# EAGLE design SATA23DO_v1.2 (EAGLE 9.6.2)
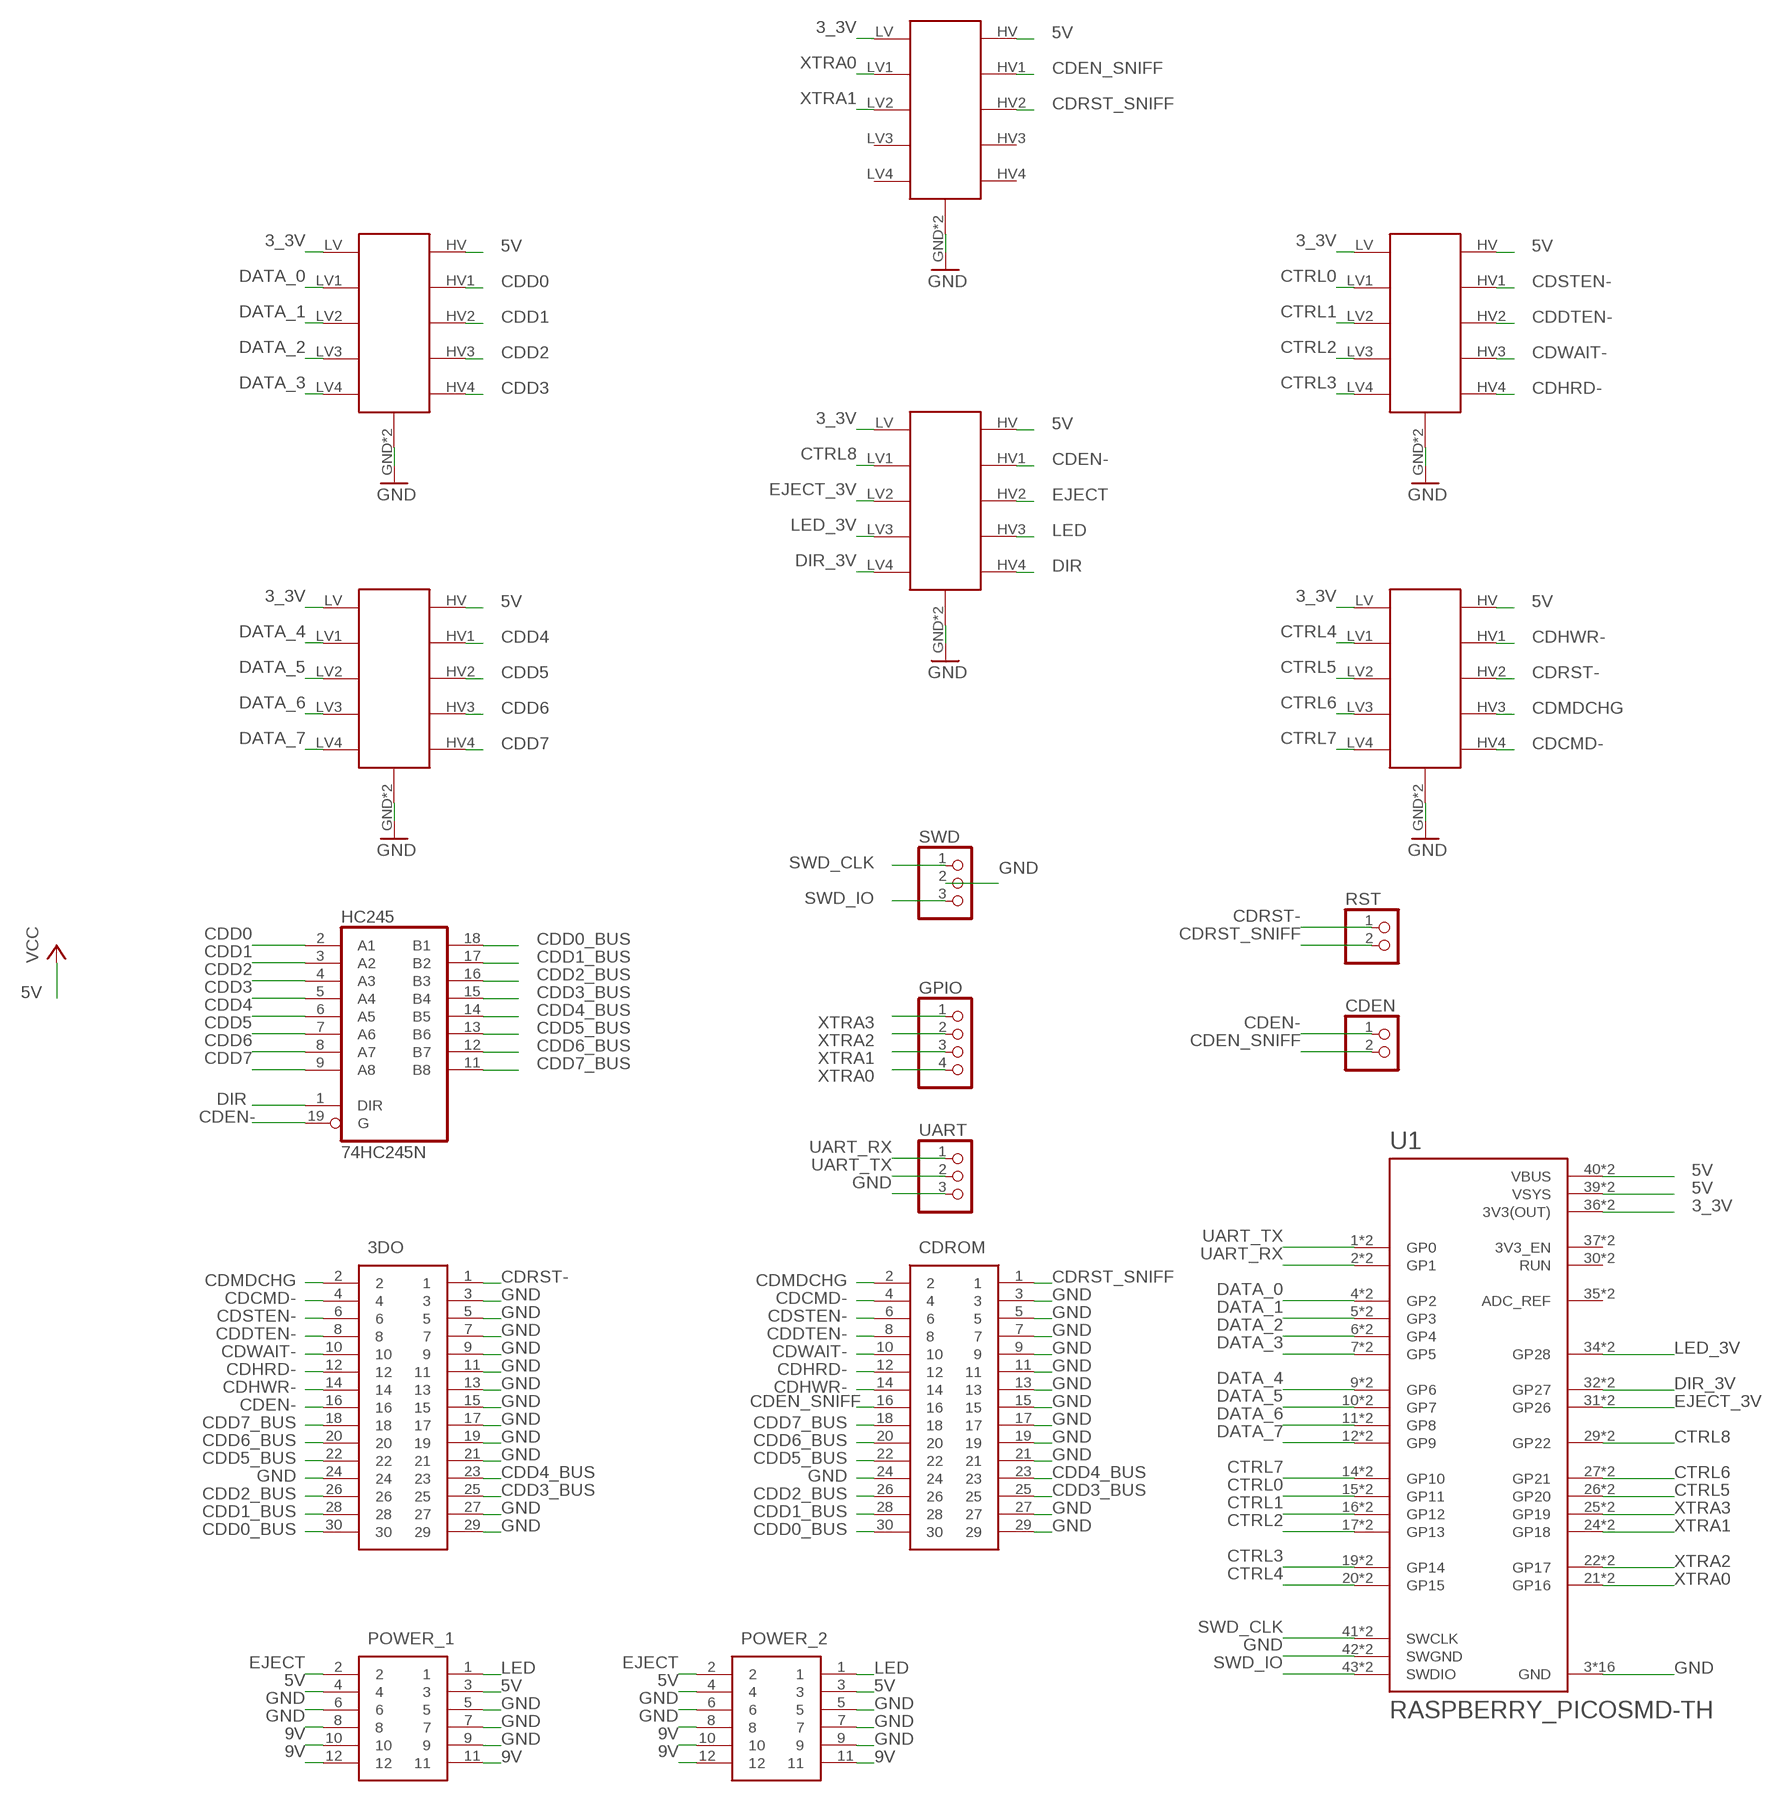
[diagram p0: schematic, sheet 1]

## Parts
3DO  52045-304530PIN_REVERSE  [30PINFFC125_REVERSE]
CDEN  PINHD-1X2  [1X02]
CDROM  52045-304530PIN_REVERSE  [30PINFFC125_REVERSE]
GPIO  PINHD-1X4  [1X04]
HC245  74HC245N  [DIL20]
POWER_1  39-53-2125  [39532125]
POWER_2  39-53-2125  [39532125]
RST  PINHD-1X2  [1X02]
SWD  PINHD-1X3  [1X03]
U1  RASPBERRY_PICOSMD-TH  [PICO-PKG]
U$1  4WAYS_LEVEL_SHIFTER  [4WAYS_LEVEL_SHIFTER]
U$5  4WAYS_LEVEL_SHIFTER  [4WAYS_LEVEL_SHIFTER]
U$6  4WAYS_LEVEL_SHIFTER  [4WAYS_LEVEL_SHIFTER]
U$7  4WAYS_LEVEL_SHIFTER  [4WAYS_LEVEL_SHIFTER]
U$8  4WAYS_LEVEL_SHIFTER  [4WAYS_LEVEL_SHIFTER]
U$9  4WAYS_LEVEL_SHIFTER  [4WAYS_LEVEL_SHIFTER]
UART  PINHD-1X3  [1X03]

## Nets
3_3V: U1.36(3V3(OUT)) U1.P$36(3V3(OUT)) U$1.LV U$5.LV U$6.LV U$7.LV U$8.LV U$9.LV
5V: POWER_1.3 POWER_1.4 POWER_2.3 POWER_2.4 U1.39(VSYS) U1.40(VBUS) U1.P$39(VSYS) U1.P$40(VBUS) U$1.HV U$5.HV U$6.HV U$7.HV U$8.HV U$9.HV ; supply symbol labelled VCC
9V: POWER_1.10 POWER_1.11 POWER_1.12 POWER_2.10 POWER_2.11 POWER_2.12
CDCMD-: 3DO.4 CDROM.4 U$7.HV4
CDD0: HC245.2(A1) U$6.HV1
CDD0_BUS: 3DO.30 CDROM.30 HC245.18(B1)
CDD1: HC245.3(A2) U$6.HV2
CDD1_BUS: 3DO.28 CDROM.28 HC245.17(B2)
CDD2: HC245.4(A3) U$6.HV3
CDD2_BUS: 3DO.26 CDROM.26 HC245.16(B3)
CDD3: HC245.5(A4) U$6.HV4
CDD3_BUS: 3DO.25 CDROM.25 HC245.15(B4)
CDD4: HC245.6(A5) U$5.HV1
CDD4_BUS: 3DO.23 CDROM.23 HC245.14(B5)
CDD5: HC245.7(A6) U$5.HV2
CDD5_BUS: 3DO.22 CDROM.22 HC245.13(B6)
CDD6: HC245.8(A7) U$5.HV3
CDD6_BUS: 3DO.20 CDROM.20 HC245.12(B7)
CDD7: HC245.9(A8) U$5.HV4
CDD7_BUS: 3DO.18 CDROM.18 HC245.11(B8)
CDDTEN-: 3DO.8 CDROM.8 U$8.HV2
CDEN-: 3DO.16 CDEN.1 HC245.19(G) U$9.HV1
CDEN_SNIFF: CDEN.2 CDROM.16 U$1.HV1
CDHRD-: 3DO.12 CDROM.12 U$8.HV4
CDHWR-: 3DO.14 CDROM.14 U$7.HV1
CDMDCHG: 3DO.2 CDROM.2 U$7.HV3
CDRST-: 3DO.1 RST.1 U$7.HV2
CDRST_SNIFF: CDROM.1 RST.2 U$1.HV2
CDSTEN-: 3DO.6 CDROM.6 U$8.HV1
CDWAIT-: 3DO.10 CDROM.10 U$8.HV3
CTRL0: U1.15(GP11) U1.P$15(GP11) U$8.LV1
CTRL1: U1.16(GP12) U1.P$16(GP12) U$8.LV2
CTRL2: U1.17(GP13) U1.P$17(GP13) U$8.LV3
CTRL3: U1.19(GP14) U1.P$19(GP14) U$8.LV4
CTRL4: U1.20(GP15) U1.P$20(GP15) U$7.LV1
CTRL5: U1.26(GP20) U1.P$26(GP20) U$7.LV2
CTRL6: U1.27(GP21) U1.P$27(GP21) U$7.LV3
CTRL7: U1.14(GP10) U1.P$14(GP10) U$7.LV4
CTRL8: U1.29(GP22) U1.P$29(GP22) U$9.LV1
DATA_0: U1.4(GP2) U1.P$4(GP2) U$6.LV1
DATA_1: U1.5(GP3) U1.P$5(GP3) U$6.LV2
DATA_2: U1.6(GP4) U1.P$6(GP4) U$6.LV3
DATA_3: U1.7(GP5) U1.P$7(GP5) U$6.LV4
DATA_4: U1.9(GP6) U1.P$9(GP6) U$5.LV1
DATA_5: U1.10(GP7) U1.P$10(GP7) U$5.LV2
DATA_6: U1.11(GP8) U1.P$11(GP8) U$5.LV3
DATA_7: U1.12(GP9) U1.P$12(GP9) U$5.LV4
DIR: HC245.1(DIR) U$9.HV4
DIR_3V: U1.32(GP27) U1.P$32(GP27) U$9.LV4
EJECT: POWER_1.2 POWER_2.2 U$9.HV2
EJECT_3V: U1.31(GP26) U1.P$31(GP26) U$9.LV2
GND: 3DO.3 3DO.5 3DO.7 3DO.9 3DO.11 3DO.13 3DO.15 3DO.17 3DO.19 3DO.21 3DO.24 3DO.27 3DO.29 CDROM.3 CDROM.5 CDROM.7 CDROM.9 CDROM.11 CDROM.13 CDROM.15 CDROM.17 CDROM.19 CDROM.21 CDROM.24 CDROM.27 CDROM.29 POWER_1.5 POWER_1.6 POWER_1.7 POWER_1.8 POWER_1.9 POWER_2.5 POWER_2.6 POWER_2.7 POWER_2.8 POWER_2.9 SWD.2 U1.3(GND) U1.8(GND) U1.13(GND) U1.18(GND) U1.23(GND) U1.28(GND) U1.33(GND) U1.38(GND) U1.42(SWGND) U1.P$3(GND) U1.P$8(GND) U1.P$13(GND) U1.P$18(GND) U1.P$23(GND) U1.P$28(GND) U1.P$33(GND) U1.P$38(GND) U1.P$42(SWGND) U$1.GND U$1.GND_1(GND) U$5.GND U$5.GND_1(GND) U$6.GND U$6.GND_1(GND) U$7.GND U$7.GND_1(GND) U$8.GND U$8.GND_1(GND) U$9.GND U$9.GND_1(GND) UART.3
LED: POWER_1.1 POWER_2.1 U$9.HV3
LED_3V: U1.34(GP28) U1.P$34(GP28) U$9.LV3
SWD_CLK: SWD.1 U1.41(SWCLK) U1.P$41(SWCLK)
SWD_IO: SWD.3 U1.43(SWDIO) U1.P$43(SWDIO)
UART_RX: U1.2(GP1) U1.P$2(GP1) UART.1
UART_TX: U1.1(GP0) U1.P$1(GP0) UART.2
XTRA0: GPIO.4 U1.21(GP16) U1.P$21(GP16) U$1.LV1
XTRA1: GPIO.3 U1.24(GP18) U1.P$24(GP18) U$1.LV2
XTRA2: GPIO.2 U1.22(GP17) U1.P$22(GP17)
XTRA3: GPIO.1 U1.25(GP19) U1.P$25(GP19)
Unconnected: U1.30(RUN) U1.35(ADC_REF) U1.37(3V3_EN) U1.P$30(RUN) U1.P$35(ADC_REF) U1.P$37(3V3_EN) U$1.HV3 U$1.HV4 U$1.LV3 U$1.LV4

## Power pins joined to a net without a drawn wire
5V: HC245.20(VCC)
GND: HC245.10(GND)

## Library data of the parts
3DO CDROM = SamacSys_Parts:52045-3045
CDEN RST = Connector:PINHD-1X2: PIN HEADER; CATEGORY: CONNECTOR; SUB-CATEGORY: PIN-HEADER
GPIO = Connector:PINHD-1X4: PIN HEADER; CATEGORY: CONNECTOR; SUB-CATEGORY: PIN-HEADER
HC245 = 74xx-eu:74*245: Octal BUS TRANSCEIVER, 3-state
POWER_1 POWER_2 = SamacSys_Parts:39-53-2125: Molex FFC/FPC THROUGH HOLE Series 1.25mm Pitch 12 Way 1 Row Straight Through Hole Female FPC Connector Source: Datasheet; ALLIED_NUMBER: 70373145; DESCRIPTION: Molex FFC/FPC THROUGH HOLE Series 1.25mm Pitch 12 Way 1 Row Straight Through Hole Female FPC Connector; HEIGHT: 10mm; MANUFACTURER_NAME: Molex; MANUFACTURER_PART_NUMBER: 39-53-2125; RS_PART_NUMBER: 5427084; RS_PRICE-STOCK: https://uk.rs-online.com/web/p/products/5427084
SWD UART = Connector:PINHD-1X3: PIN HEADER; CATEGORY: CONNECTOR; SUB-CATEGORY: PIN-HEADER
U1 = RpiPico:RASPBERRY_PICO: Raspberry Pi Pico
U$1 U$5-U$9 = FunModules:4WAYS_LEVEL_SHIFTER

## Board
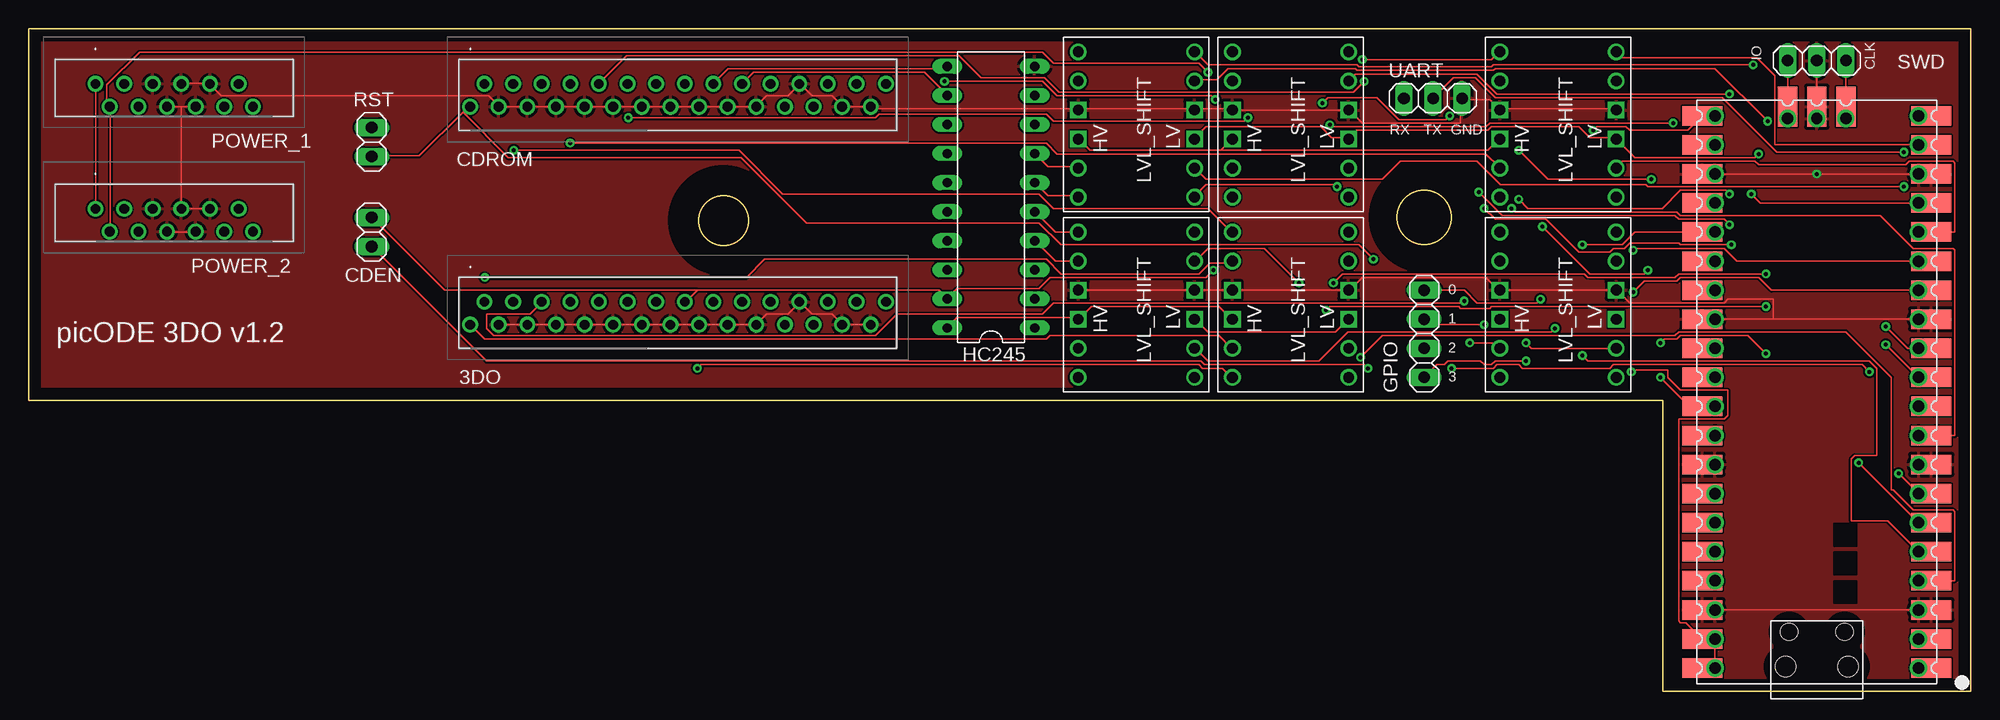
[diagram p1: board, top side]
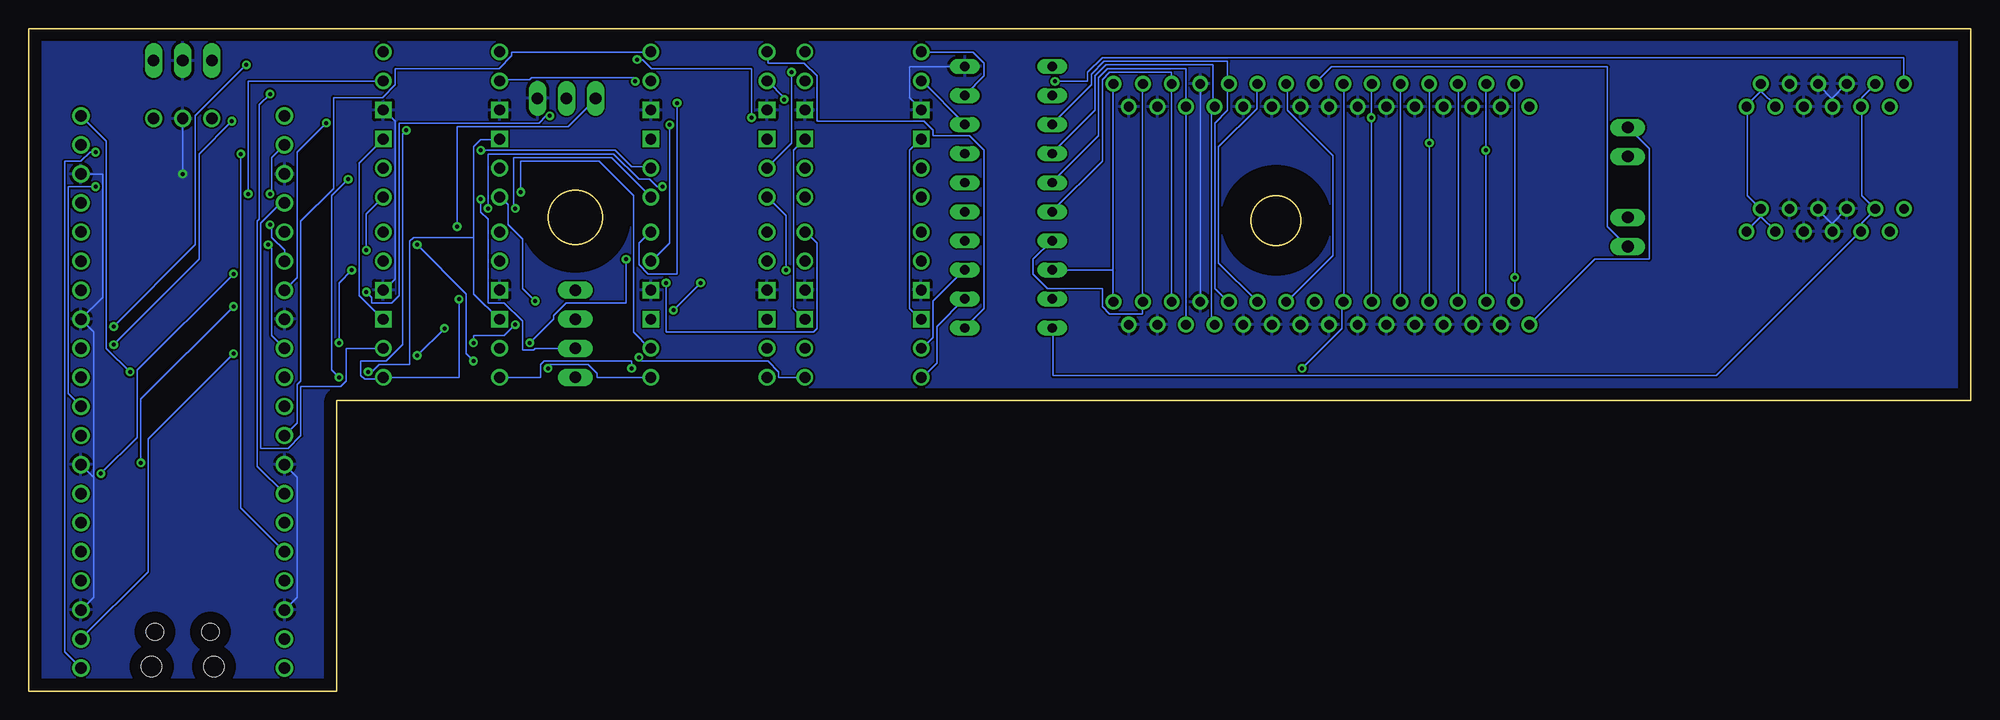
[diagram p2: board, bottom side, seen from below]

Size 169.67 x 57.91 mm. Coordinates in mm from the lower left corner, seen from the top.
Outline: 0,25.4 0,57.91 169.67,57.91 169.67,0 142.75,0 142.75,25.4 0,25.4
Outline: circle at 60.71,41.15 radius 2.16
Outline: circle at 121.92,41.4 radius 2.34
Copper layers (1*16): Top 0.035mm / dielectric 1.5mm / Bottom 0.035mm
Design rules "default": minimum track width 6mil, minimum drill 0.35mm, track to track 6mil, track to pad 6mil, pad to pad 6mil, via to via 6mil, smd to smd 6mil, copper to edge 40mil, drill to drill 6mil, minimum pad ring 10mil, minimum via ring 8mil, stop-mask expansion 4mil, vias tented up to drill 0mil, thermal gap 10mil
tRestrict: area 118.4,37.8 to 125.5,45; area 57.2,37.6 to 64.3,44.7
bRestrict: area 118.4,37.8 to 125.5,45; area 57.2,37.6 to 64.3,44.7

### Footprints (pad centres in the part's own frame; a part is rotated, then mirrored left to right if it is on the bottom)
30PINFFC125_REVERSE = drill 0.85 pad 1.381: 1 -5.12,-0.73; 2 -3.87,1.27; 3 -2.62,-0.73; 4 -1.37,1.27; 5 -0.12,-0.73; 6 1.13,1.27; 7 2.38,-0.73; 8 3.63,1.27; 9 4.88,-0.73; 10 6.13,1.27; 11 7.38,-0.73; 12 8.63,1.27; 13 9.88,-0.73; 14 11.13,1.27; 15 12.38,-0.73; 16 13.63,1.27; 17 14.88,-0.73; 18 16.13,1.27; 19 17.38,-0.73; 20 18.63,1.27; 21 19.88,-0.73; 22 21.13,1.27; 23 22.38,-0.73; 24 23.63,1.27; 25 24.88,-0.73; 26 26.13,1.27; 27 27.38,-0.73; 28 28.63,1.27; 29 29.88,-0.73; 30 31.222,1.27
1X02 = drill 1.016 long: 1 -1.27,0; 2 1.27,0
1X04 = drill 1.016 long: 1 -3.81,0; 2 -1.27,0; 3 1.27,0; 4 3.81,0
DIL20 = drill 0.813 long: 1 -11.43,-3.81; 2 -8.89,-3.81; 3 -6.35,-3.81; 4 -3.81,-3.81; 5 -1.27,-3.81; 6 1.27,-3.81; 7 3.81,-3.81; 8 6.35,-3.81; 9 8.89,-3.81; 10 11.43,-3.81; 11 11.43,3.81; 12 8.89,3.81; 13 6.35,3.81; 14 3.81,3.81; 15 1.27,3.81; 16 -1.27,3.81; 17 -3.81,3.81; 18 -6.35,3.81; 19 -8.89,3.81; 20 -11.43,3.81
39532125 = drill 0.85 pad 1.381: 1 0,0; 2 1.25,-2; 3 2.5,0; 4 3.75,-2; 5 5,0; 6 6.25,-2; 7 7.5,0; 8 8.75,-2; 9 10,0; 10 11.25,-2; 11 12.5,0; 12 13.75,-2
1X03 = drill 1.016 long: 1 -2.54,0; 2 0,0; 3 2.54,0
PICO-PKG = drill 1: 1 -8.89,24.13; 2 -8.89,21.59; 3 -8.89,19.05; 4 -8.89,16.51; 5 -8.89,13.97; 6 -8.89,11.43; 7 -8.89,8.89; 8 -8.89,6.35; 9 -8.89,3.81; 10 -8.89,1.27; 11 -8.89,-1.27; 12 -8.89,-3.81; 13 -8.89,-6.35; 14 -8.89,-8.89; 15 -8.89,-11.43; 16 -8.89,-13.97; 17 -8.89,-16.51; 18 -8.89,-19.05; 19 -8.89,-21.59; 20 -8.89,-24.13; 21 8.89,-24.13; 22 8.89,-21.59; 23 8.89,-19.05; 24 8.89,-16.51; 25 8.89,-13.97; 26 8.89,-11.43; 27 8.89,-8.89; 28 8.89,-6.35; 29 8.89,-3.81; 30 8.89,-1.27; 31 8.89,1.27; 32 8.89,3.81; 33 8.89,6.35; 34 8.89,8.89; 35 8.89,11.43; 36 8.89,13.97; 37 8.89,16.51; 38 8.89,19.05; 39 8.89,21.59; 40 8.89,24.13; 41 -2.54,-23.9; 42 0,-23.9; 43 2.54,-23.9 | smd 3.5 x 1.7: P$1 -10,24.13; P$2 -10,21.59; P$3 -10,19.05; P$4 -10,16.51; P$5 -10,13.97; P$6 -10,11.43; P$7 -10,8.89; P$8 -10,6.35; P$9 -10,3.81; P$10 -10,1.27; P$11 -10,-1.27; P$12 -10,-3.81; P$13 -10,-6.35; P$14 -10,-8.89; P$15 -10,-11.43; P$16 -10,-13.97; P$17 -10,-16.51; P$18 -10,-19.05; P$19 -10,-21.59; P$20 -10,-24.13; P$21 10,-24.13; P$22 10,-21.59; P$23 10,-19.05; P$24 10,-16.51; P$25 10,-13.97; P$26 10,-11.43; P$27 10,-8.89; P$28 10,-6.35; P$29 10,-3.81; P$30 10,-1.27; P$31 10,1.27; P$32 10,3.81; P$33 10,6.35; P$34 10,8.89; P$35 10,11.43; P$36 10,13.97; P$37 10,16.51; P$38 10,19.05; P$39 10,21.59; P$40 10,24.13 | smd 1.7 x 3.5: P$41 -2.54,-24.925; P$42 0,-24.925; P$43 2.54,-24.925 | hole 1.8: -2.725,24; 2.725,24 | hole 1.5: -2.425,20.97; 2.425,20.97
4WAYS_LEVEL_SHIFTER = drill 0.95 square: GND -5.08,-1.27; GND_1 5.08,-1.27; HV 5.08,1.27; LV -5.08,1.27 | drill 0.95: HV1 5.08,6.35; HV2 5.08,3.81; HV3 5.08,-3.81; HV4 5.08,-6.35; LV1 -5.08,6.35; LV2 -5.08,3.81; LV3 -5.08,-3.81; LV4 -5.08,-6.35

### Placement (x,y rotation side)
3DO  43.69,32.77 0 top
CDEN  29.97,40.13 270 top
CDROM  43.69,51.82 0 top
GPIO  121.92,31.24 90 top
HC245  84.07,43.18 90 top
POWER_1  5.84,53.09 0 top
POWER_2  5.84,42.16 0 top
RST  29.97,48.01 270 top
SWD  156.21,55.12 180 top
U1  156.21,26.16 180 top
U$1  133.6,33.78 180 top
U$5  96.77,49.53 180 top
U$6  96.77,33.78 180 top
U$7  110.24,33.78 180 top
U$8  133.6,49.53 180 top
U$9  110.24,49.53 180 top
UART  122.68,51.82 0 top

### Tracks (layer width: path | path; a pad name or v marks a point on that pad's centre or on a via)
3_3V  (via drill 0.35)
  Top 0.152: U$6.LV 101.92,32.51 103.03,31.4 114.14,31.4 115.25,32.51 U$7.LV | U$5.LV 101.92,48.39 102.87,49.34 112.87,49.34 113.82,48.39 115.25,48.39 U$9.LV 115.41,48.39 116.05,49.02 127.48,49.02 127.79,49.34 135.41,49.34 136.37,48.39 138.59,48.39 U$8.LV 138.75,48.23 140.34,46.64 150.81,46.64 v151.13,46.96 | U1.P$36 U1.36
  Bottom 0.152: U$6.LV 101.92,32.51 102.87,33.46 102.87,47.28 101.92,48.23 U$5.LV | U$1.LV 138.75,32.51 140.81,34.58 140.81,46.16 138.75,48.23 U$8.LV | U1.36 151.13,16 v151.13,46.96
5V  (via drill 0.35)
  Top 0.152: U1.P$40 U1.40 U1.39 U1.P$39 144.78,6 144.3,6 144.15,6.16 144.15,23.78 148.11,23.78 148.43,24.1 148.43,26.32 144.3,26.32 143.19,27.43 143.19,28.07 140.18,28.07 v140.02,27.91 | 104.14,47.28 92.71,47.28 91.76,48.23 U$5.HV | 104.14,47.28 105.09,48.23 U$9.HV | HC245.20 80.33,31.88 81.12,32.67 91.44,32.67 91.6,32.51 U$6.HV 91.76,32.51 92.87,33.62 103.98,33.62 105.09,32.51 U$7.HV | 104.14,47.28 127.48,47.28 128.43,48.23 U$8.HV
  Bottom 0.152: 130.81,39.66 130.81,47.59 130.18,48.23 128.59,48.23 U$8.HV | 130.81,39.66 130.81,34.73 128.59,32.51 U$1.HV | v140.02,27.91 139.7,27.91 139.06,28.54 136.37,28.54 136.37,39.34 136.05,39.66 130.81,39.66 | POWER_1.3 8.41,52.99 9.53,51.88 9.53,51.24 POWER_1.4 9.53,51.09 9.53,43.31 8.41,42.2 POWER_2.3 8.41,42.04 9.53,40.93 9.53,40.29 POWER_2.4 9.68,40.13 22.23,27.59 80.17,27.59 80.17,31.72 HC245.20 | U$5.HV 91.76,48.23 92.71,47.28 92.71,33.46 91.76,32.51 U$6.HV
9V
  Bottom 0.152: 18.26,41.56 18.26,42.04 POWER_2.11 | 18.26,41.56 18.26,41.4 17.14,40.29 POWER_2.10 | 18.26,41.56 19.53,40.29 POWER_2.12 | 18.26,41.56 POWER_2.11 | 18.26,52.51 18.26,52.99 POWER_1.11 18.26,52.51 | 18.26,52.51 18.26,52.36 17.14,51.24 POWER_1.10 | 18.26,52.51 19.53,51.24 POWER_1.12 19.53,51.09 19.53,43.31 18.41,42.2 POWER_2.11
CDCMD-  (via drill 0.35)
  Top 0.152: v42.39,47.28 62.07,47.28 65.88,43.47 88.27,43.47 89.53,42.2 103.03,42.2 105.09,40.13 U$7.HV4
  Bottom 0.152: 3DO.4 42.39,34.1 v42.39,47.28 42.39,52.99 CDROM.4
CDD0
  Bottom 0.152: HC245.2 87.95,34.26 90.33,31.88 90.33,28.7 91.6,27.43 U$6.HV1
CDD0_BUS
  Bottom 0.152: 74.93,36.8 80.17,36.8 HC245.18 | 74.93,36.8 74.93,34.1 3DO.30 | 74.93,36.8 74.93,52.99 CDROM.30
CDD1
  Bottom 0.152: HC245.3 87.95,36.8 90.65,34.1 90.65,30.92 91.6,29.97 U$6.HV2
CDD1_BUS
  Bottom 0.152: HC245.17 80.33,39.34 81.92,37.75 81.92,36.48 80.64,35.21 75.88,35.21 75.88,33.62 75.25,32.99 72.39,32.99 72.39,33.94 3DO.28 72.39,34.1 72.39,52.99 CDROM.28
CDD2
  Top 0.152: U$6.HV3 89.69,37.59 87.95,39.34 HC245.4
CDD2_BUS
  Bottom 0.152: HC245.16 80.17,42.04 75.88,46.32 75.88,53.47 75.25,54.1 69.85,54.1 69.85,53.15 CDROM.26 69.85,52.99 69.85,34.1 3DO.26
CDD3
  Top 0.152: U$6.HV4 89.69,40.13 87.95,41.88 HC245.5
CDD3_BUS
  Bottom 0.152: HC245.15 80.17,44.58 76.2,48.55 76.2,53.63 75.41,54.42 68.58,54.42 68.58,51.24 CDROM.25 68.58,32.2 3DO.25
CDD4
  Top 0.152: HC245.6 87.95,44.42 89.06,43.31 91.6,43.31 U$5.HV1
CDD4_BUS
  Bottom 0.152: HC245.14 80.17,47.12 76.52,50.77 76.52,53.79 75.56,54.74 66.2,54.74 66.2,51.24 CDROM.23 66.2,51.09 66.36,50.93 66.36,32.35 66.2,32.2 3DO.23
CDD5
  Top 0.152: HC245.7 87.95,46.96 89.06,45.85 91.6,45.85 U$5.HV2
CDD5_BUS
  Bottom 0.152: HC245.13 80.17,49.66 76.83,52.99 76.83,53.94 75.72,55.05 64.93,55.05 64.93,53.15 CDROM.22 64.93,52.99 64.93,50.77 66.04,49.66 66.04,35.21 64.93,34.1 3DO.22
CDD6
  Bottom 0.152: HC245.8 87.95,49.66 91.6,53.31 U$5.HV3
CDD6_BUS
  Top 0.152: HC245.12 80.17,52.2 78.26,54.1 63.34,54.1 62.39,53.15 CDROM.20
  Bottom 0.152: 3DO.20 62.39,34.1 65.72,37.43 65.72,47.59 62.39,50.93 62.39,52.99 CDROM.20
CDD7
  Bottom 0.152: HC245.9 87.79,52.2 86.2,53.79 86.2,54.9 87.15,55.85 91.6,55.85 U$5.HV4
CDD7_BUS
  Top 0.152: HC245.11 80.17,54.58 80.01,54.42 61.12,54.42 59.85,53.15 CDROM.18
  Bottom 0.152: 3DO.18 59.69,34.1 55.72,38.07 55.72,46.8 59.69,50.77 59.69,52.99 CDROM.18
CDDTEN-  (via drill 0.35)
  Top 0.152: v47.31,47.91 88.9,47.91 89.85,46.96 127.32,46.96 128.43,45.85 U$8.HV2
  Bottom 0.152: 3DO.8 47.31,34.1 v47.31,47.91 47.31,52.99 CDROM.8
CDEN-  (via drill 0.35)
  Top 0.152: 58.42,35.05 79.53,35.05 80.17,34.42 HC245.19 80.33,34.42 81.12,35.21 88.27,35.21 89.22,36.16 102.87,36.16 v103.5,36.8 | 58.42,35.05 57.47,34.1 3DO.16 | 58.42,35.05 36.35,35.05 30,41.4 CDEN.1
  Bottom 0.152: v103.5,36.8 103.5,41.56 105.09,43.15 U$9.HV1
CDEN_SNIFF  (via drill 0.35)
  Top 0.152: v117,28.23 116.68,28.54 102.71,28.54 102.39,28.86 40.01,28.86 30,38.86 CDEN.2
  Bottom 0.152: CDROM.16 57.31,53.15 55.88,54.58 31.75,54.58 31.75,40.61 30,38.86 CDEN.2 | U$1.HV1 124.94,27.43 124.94,28.54 124.62,28.86 117,28.86 v117,28.23
CDHRD-  (via drill 0.35)
  Top 0.152: v116.52,55.21 127.79,55.21 128.43,55.85 U$8.HV4 | v106.52,50.13 106.2,49.82 89.53,49.82 88.9,50.45 74.3,50.45 73.98,50.13 v52.39,50.13
  Bottom 0.152: 3DO.12 52.39,34.1 v52.39,50.13 52.39,52.99 CDROM.12 | v116.52,55.21 116.05,55.21 115.25,54.42 106.52,54.42 v106.52,50.13
CDHWR-  (via drill 0.35)
  Top 0.152: v58.42,28.23 58.74,28.54 102.23,28.54 102.55,28.23 104.3,28.23 105.09,27.43 U$7.HV1
  Bottom 0.152: CDROM.14 54.77,52.99 54.77,34.1 3DO.14 54.93,33.94 54.93,31.72 v58.42,28.23
CDMDCHG  (via drill 0.35)
  Top 0.152: v39.85,36.16 62.71,36.16 64.29,37.75 88.9,37.75 90.17,36.48 102.23,36.48 103.19,37.43 104.93,37.43 105.09,37.59 U$7.HV3
  Bottom 0.152: 3DO.2 39.85,34.1 v39.85,36.16 39.85,52.99 CDROM.2
CDRST-
  Top 0.152: U$7.HV2 105.09,29.97 103.98,31.08 89.22,31.08 88.9,30.77 39.85,30.77 3DO.1
  Bottom 0.152: 3DO.1 38.42,32.2 32.86,37.75 28.1,37.75 28.1,47.43 29.84,49.18 RST.1
CDRST_SNIFF  (via drill 0.35)
  Top 0.152: 37.94,50.61 34.13,46.8 30,46.8 RST.2 | 37.94,50.61 38.42,51.09 CDROM.1 | v125.89,30.45 127.95,30.45 128.43,29.97 U$1.HV2 | v117.47,37.75 116.2,39.02 90.17,39.02 88.27,40.93 67.94,40.93 62.23,46.64 41.91,46.64 37.94,50.61
  Bottom 0.152: v125.89,30.45 123.83,32.51 123.83,32.83 122.71,33.94 117.47,33.94 v117.47,37.75
CDSTEN-  (via drill 0.35)
  Top 0.152: v125.41,34.1 125.25,33.94 89.53,33.94 88.58,32.99 75.88,32.99 73.98,31.08 40.64,31.08 40.01,31.72 40.01,32.99 43.81,32.99 44.77,33.94 3DO.6
  Bottom 0.152: 3DO.6 44.77,34.1 44.77,52.99 CDROM.6 | v125.41,34.1 126.52,35.21 126.52,39.5 127.79,40.77 127.79,42.51 128.43,43.15 U$8.HV1
CDWAIT-  (via drill 0.35)
  Top 0.152: v116.68,53.31 115.73,52.36 90.01,52.36 88.74,53.63 83.19,53.63 81.28,55.53 52.23,55.53 49.85,53.15 CDROM.10
  Bottom 0.152: 3DO.10 49.85,34.1 49.85,52.99 CDROM.10 | v116.68,53.31 116.68,53.63 125.73,53.63 125.89,53.47 128.43,53.47 U$8.HV3
CTRL0  (via drill 0.35)
  Top 0.152: v140.18,38.54 140.34,38.7 148.11,38.7 149.22,37.59 U1.15 U1.P$15
  Bottom 0.152: v140.18,38.54 140.18,41.72 138.75,43.15 U$8.LV1
CTRL1
  Top 0.152: U$8.LV2 138.75,45.85 139.22,46.32 150.81,46.32 151.13,46.01 163.99,46.01 164.31,46.32 168.12,46.32 168.28,46.16 168.28,40.13 U1.P$16 U1.16
CTRL2  (via drill 0.35)
  Top 0.152: v150.5,43.47 151.29,42.67 U1.17 U1.P$17
  Bottom 0.152: v150.5,43.47 150.5,53.31 138.75,53.31 U$8.LV3
CTRL3
  Top 0.152: U$8.LV4 138.75,55.85 139.22,55.37 150.97,55.37 152.56,53.79 152.56,47.75 U1.19 U1.P$19
CTRL4  (via drill 0.35)
  Top 0.152: v124.3,28.23 127.95,28.23 128.27,28.54 130.18,28.54 130.49,28.23 138.11,28.23 138.43,28.54 160.18,28.54 v160.81,27.91 | U1.20 U1.P$20
  Bottom 0.152: U$7.LV1 120.02,27.43 120.02,27.75 120.81,28.54 124.3,28.54 v124.3,28.23 | v160.81,27.91 162.88,29.97 162.88,48.07 U1.20
CTRL5  (via drill 0.35)
  Top 0.152: v126.68,43.62 128.75,41.56 143.83,41.56 144.15,41.24 148.11,41.24 v148.59,40.77 | U1.26 U1.P$26
  Bottom 0.152: v126.68,43.62 126.68,46.32 119.86,46.32 116.84,43.31 116.84,31.4 115.41,29.97 U$7.LV2 | v148.59,40.77 148.43,40.61 148.43,39.66 147.32,38.54 U1.26
CTRL6  (via drill 0.35)
  Top 0.152: v113.67,49.5 113.82,49.34 127.32,49.34 127.64,49.66 v143.67,49.66 | U1.27 U1.P$27
  Bottom 0.152: v113.67,49.5 113.67,39.18 115.25,37.59 U$7.LV3 | v143.67,49.66 146.21,47.12 146.21,36.16 U1.27
CTRL7  (via drill 0.35)
  Top 0.152: v113.03,51.4 113.51,51.88 117.79,51.88 119.7,49.98 123.83,49.98 v124.14,50.29 | v140.18,34.89 141.13,35.85 143.99,35.85 144.3,36.16 151.13,36.16 152.24,35.05 U1.14 U1.P$14
  Bottom 0.152: v113.03,51.4 113.03,36.48 115.57,36.48 116.36,37.27 116.36,39.18 115.41,40.13 U$7.LV4 | v124.14,50.29 124.46,50.29 125.09,49.66 137.32,49.66 137.32,34.58 137.95,33.94 139.7,33.94 139.7,34.42 v140.18,34.89
CTRL8  (via drill 0.35)
  Top 0.152: v127.16,42.2 128.11,41.24 132.56,41.24 135.41,38.39 138.11,38.39 138.43,38.7 139.38,38.7 139.86,39.18 144.15,39.18 144.3,39.02 v148.75,39.02 | U1.29 U1.P$29
  Bottom 0.152: v127.16,42.2 127.32,42.35 127.32,46.64 118.75,46.64 115.41,43.31 U$9.LV1 | v148.75,39.02 148.43,38.7 148.43,31.08 U1.29
DATA_0  (via drill 0.35)
  Top 0.152: v116.36,29.18 118.27,31.08 143.83,31.08 144.15,31.4 158.75,31.4 162.72,27.43 162.72,17.59 162.88,17.59 164.62,15.84 168.12,15.84 168.28,15.68 168.28,9.65 U1.P$4 U1.4
  Bottom 0.152: U$6.LV1 104.14,27.43 104.14,27.91 105.09,28.86 116.36,28.86 v116.36,29.18
DATA_1  (via drill 0.35)
  Top 0.152: v133.35,31.72 133.03,31.4 115.25,31.4 112.71,28.86 103.03,28.86 101.92,29.97 U$6.LV2 | v135.73,29.34 136.21,28.86 160.81,28.86 161.45,28.23 161.45,20.61 159.54,20.61 159.23,20.29 159.23,14.89 162.4,14.89 U1.5 U1.P$5
  Bottom 0.152: v135.73,29.34 v133.35,31.72
DATA_2  (via drill 0.35)
  Top 0.152: v110.97,35.69 107.95,38.7 103.03,38.7 101.92,37.59 U$6.LV3 | v113.35,33.31 113.67,33.62 124.94,33.62 125.09,33.46 127.64,33.46 127.79,33.62 v151.76,33.62 | v159.86,19.97 U1.6 U1.P$6
  Bottom 0.152: v113.35,33.31 v110.97,35.69 | v151.76,33.62 159.86,25.53 v159.86,19.97
DATA_3  (via drill 0.35)
  Top 0.152: v113.98,35.69 114.78,36.48 135.89,36.48 136.21,36.16 143.83,36.16 144.15,36.48 v151.76,36.48 | v163.35,19.02 U1.7 U1.P$7
  Bottom 0.152: v113.98,35.69 113.98,31.4 101.12,31.4 100.81,31.72 100.81,39.18 101.76,40.13 U$6.LV4 | v151.76,36.48 160.18,28.07 160.18,22.19 v163.35,19.02
DATA_4  (via drill 0.35)
  Top 0.152: v114.3,44.1 114.14,44.26 102.87,44.26 101.92,43.31 U$5.LV1 | v129.54,42.2 129.86,41.88 143.99,41.88 144.3,41.56 161.77,41.56 164.62,38.7 168.12,38.7 168.28,38.54 168.28,22.35 U1.P$9 U1.9
  Bottom 0.152: v114.3,44.1 114.78,44.1 115.41,44.74 116.36,44.74 118.59,46.96 129.54,46.96 v129.54,42.2
DATA_5  (via drill 0.35)
  Top 0.152: v163.83,44.1 141.45,44.1 141.29,44.26 128.59,44.26 126.52,46.32 119.86,46.32 118.27,44.74 102.87,44.74 101.92,45.69 U$5.LV2 | U1.10 U1.P$10
  Bottom 0.152: v163.83,44.1 166.21,44.1 166.21,26 U1.10
DATA_6  (via drill 0.35)
  Top 0.152: v151.92,49.82 147.32,54.42 128.11,54.42 127.95,54.26 116.05,54.26 115.89,54.42 104.78,54.42 103.82,53.47 101.92,53.47 U$5.LV3 | v162.24,30.29 U1.11 U1.P$11
  Bottom 0.152: v151.92,49.82 154.78,46.96 154.78,37.75 v162.24,30.29
DATA_7  (via drill 0.35)
  Top 0.152: v150.65,54.74 127.95,54.74 127.79,54.58 116.2,54.58 116.05,54.74 103.03,54.74 101.92,55.85 U$5.LV4 | v162.24,31.88 164.15,29.97 U1.12 U1.P$12
  Bottom 0.152: v150.65,54.74 155.1,50.29 155.1,39.02 v162.24,31.88
DIR
  Bottom 0.152: HC245.1 87.79,31.88 86.2,33.46 86.2,47.28 87.47,48.55 90.65,48.55 90.65,49.02 91.44,49.82 100.81,49.82 100.81,53.79 101.92,54.9 105.09,54.9 105.09,55.85 U$9.HV4
DIR_3V
  Top 0.152: U1.32 U1.P$32
  Bottom 0.152: U1.32 146.21,23.46 146.21,26.8 145.89,27.12 145.89,41.09 143.03,43.94 143.03,51.88 138.75,51.88 137.64,52.99 137.64,54.42 128.59,54.42 127.48,55.53 127.48,55.85 115.41,55.85 U$9.LV4
EJECT  (via drill 0.35)
  Top 0.152: POWER_2.2 7.14,40.29 7.14,51.09 POWER_1.2 6.99,51.24 6.83,51.24 6.83,52.99 9.68,55.85 88.58,55.85 89.53,54.9 102.23,54.9 v103.03,54.1
  Bottom 0.152: v103.03,54.1 103.03,47.91 105.09,45.85 U$9.HV2
EJECT_3V  (via drill 0.35)
  Top 0.152: v130.18,47.28 132.72,44.74 v141.76,44.74 | v142.56,27.43 145.1,24.89 U1.P$31 U1.31
  Bottom 0.152: v130.18,47.28 118.43,47.28 117,45.85 115.41,45.85 U$9.LV2 | v141.76,44.74 143.19,43.31 143.19,28.07 v142.56,27.43
GND  (via drill 0.35)
  Top 0.152: 3DO.29 73.5,32.04 71.12,32.04 3DO.27 70.96,32.2 70.17,32.99 68.42,32.99 67.47,33.94 3DO.24 67.31,33.94 66.36,32.99 64.45,32.99 63.66,32.2 3DO.21 63.5,32.04 61.12,32.04 3DO.19 60.96,32.04 3DO.17 58.42,32.04 56.2,32.04 3DO.15 56.04,32.04 53.66,32.04 3DO.13 53.5,32.04 51.12,32.04 3DO.11 50.96,32.04 3DO.9 48.42,32.04 46.2,32.04 3DO.7 46.04,32.04 43.66,32.04 3DO.5 43.5,32.04 41.12,32.04 3DO.3 | POWER_2.6 12.22,40.13 14.45,40.13 POWER_2.8 | POWER_2.9 15.72,42.2 13.49,42.2 POWER_2.7 13.34,42.2 13.34,51.09 | 13.34,51.09 14.45,51.09 POWER_1.8 | 13.34,51.09 12.22,51.09 POWER_1.6 | POWER_1.7 13.49,53.15 15.72,53.15 POWER_1.9 15.88,52.99 16.83,52.04 40.16,52.04 40.96,51.24 CDROM.3 41.12,51.09 43.5,51.09 CDROM.5 43.66,51.09 46.04,51.09 CDROM.7 46.2,51.09 48.42,51.09 CDROM.9 50.96,51.09 CDROM.11 51.12,51.09 53.5,51.09 CDROM.13 53.66,51.09 56.04,51.09 CDROM.15 56.2,51.09 58.42,51.09 CDROM.17 60.96,51.09 CDROM.19 61.12,51.09 63.5,51.09 CDROM.21 63.66,51.24 64.45,52.04 66.36,52.04 67.31,52.99 CDROM.24 67.47,52.99 68.42,52.04 70.17,52.04 70.96,51.24 CDROM.27 71.12,51.09 73.5,51.09 CDROM.29 73.66,51.09 73.82,50.93 91.6,50.93 U$5.GND_1 91.76,50.93 101.76,50.93 U$5.GND 101.92,50.93 105.09,50.93 U$9.GND_1 105.25,50.77 115.25,50.77 U$9.GND 115.41,50.77 116.52,49.66 125.09,49.66 125.09,51.72 UART.3 125.25,51.72 127.64,51.72 128.43,50.93 U$8.GND_1 128.59,50.93 138.59,50.93 U$8.GND | U1.42 U1.P$42 SWD.2 | U1.P$23 U1.23 v156.21,45.21 U1.18 U1.P$18 | U1.P$28 U1.28 152.4,32.51 | U1.P$13 U1.13 152.4,32.51 | U1.P$38 U1.38 U1.3 U1.P$3 | U1.P$33 U1.33
  Top 0.152: U1.P$8 U1.8 | U$6.GND_1 U$6.GND U$7.GND_1 U$7.GND 115.41,35.05 116.52,36.16 127.32,36.16 128.43,35.05 U$1.GND_1 U$1.GND 138.75,35.05 139.86,33.94 148.11,33.94 148.43,34.26 152.4,34.26 152.4,32.51
  Bottom 0.152: 12.06,40.77 12.06,40.29 POWER_2.6 12.06,40.77 | 12.06,40.77 12.06,40.93 10.95,42.04 POWER_2.5 | 12.06,40.77 13.34,42.04 POWER_2.7 | 12.06,51.72 12.06,51.24 POWER_1.6 12.06,51.72 | 12.06,51.72 12.06,51.88 10.95,52.99 POWER_1.5 | 12.06,51.72 13.34,52.99 POWER_1.7 | 3DO.24 67.31,34.1 67.31,52.99 CDROM.24 | v156.21,45.21 U1.42 | U1.38 146.21,8.22 146.21,18.7 U1.33 | U1.3 163.99,8.22 163.99,18.7 | U1.8 163.99,18.7 | 163.99,18.7 163.99,31.4 U1.13 163.19,34.42 163.19,45.21 U1.18 | HC245.10 87.95,54.58 92.71,54.58 92.71,51.88 91.76,50.93 U$5.GND_1 | U$1.GND 138.59,35.05 137.64,36.01 137.64,49.82 138.59,50.77 U$8.GND
  pour Top: 0,57.91 0,25.4 142.49,25.4 142.75,25.65 142.75,0.25 143,0 169.16,0 169.42,0.25 169.42,57.66 0.25,57.66
  pour Bottom: 0,57.91 0,25.91 -0.25,25.65 142.75,25.65 142.75,0 169.42,0 169.42,57.66 0.25,57.66
LED  (via drill 0.35)
  Top 0.152: POWER_2.1 5.87,42.2 5.87,52.99 POWER_1.1 | v103.66,51.72 103.35,52.04 89.85,52.04 88.58,53.31 v80.01,53.31
  Bottom 0.152: v103.66,51.72 103.66,51.88 105.09,53.31 U$9.HV3 | v80.01,53.31 77.15,53.31 77.15,54.1 75.88,55.37 5.87,55.37 5.87,53.15 POWER_1.1
LED_3V  (via drill 0.35)
  Top 0.152: v148.59,52.2 128.27,52.2 126.52,53.94 115.89,53.94 115.41,53.47 U$9.LV3 | U1.34 U1.P$34
  Bottom 0.152: v148.59,52.2 149.54,51.24 149.54,41.24 149.7,41.09 149.7,19.65 U1.34
SWD_CLK
  Top 0.152: U1.41 U1.P$41 SWD.1
SWD_IO
  Top 0.152: U1.43 U1.P$43 SWD.3
UART_RX  (via drill 0.35)
  Top 0.152: U1.P$2 U1.2 | v132.24,40.61 136.37,36.48 141.13,36.48 v141.45,36.8 | v142.56,30.45 142.88,30.77 143.99,30.77 144.3,31.08 150.18,31.08 v151.76,29.5
  Bottom 0.152: v132.24,40.61 132.24,49.34 122.56,49.34 120.17,51.72 UART.1 | v141.45,36.8 142.56,35.69 v142.56,30.45 | v151.76,29.5 159.23,22.03 159.23,10.45 U1.2
UART_TX  (via drill 0.35)
  Top 0.152: U1.P$1 U1.1 | v163.83,47.12 152.72,47.12 147.96,51.88 128.11,51.88 126.36,53.63 124.46,53.63 122.71,51.88 UART.2
  Bottom 0.152: v163.83,47.12 164.31,47.12 165.1,46.32 166.53,46.32 166.53,3.46 U1.1
XTRA0  (via drill 0.35)
  Top 0.152: U1.21 U1.P$21 144.94,49.02 139.86,49.02 139.54,49.34 137,49.34 v136.68,49.02 | v132.08,34.26 131.76,33.94 126.52,33.94 125.41,35.05 GPIO.4
  Bottom 0.152: v132.08,34.26 132.08,27.43 U$1.LV1 138.75,27.43 138.75,27.27 140.34,27.27 140.65,27.59 140.65,28.86 138.43,28.86 137,30.29 137,48.7 v136.68,49.02
XTRA1  (via drill 0.35)
  Top 0.152: GPIO.3 122.4,32.04 v127.16,32.04 | v130.81,30.45 131.29,29.97 U$1.LV2 | U1.24 U1.P$24
  Bottom 0.152: U$1.LV2 141.92,29.97 141.92,27.12 142.4,26.64 145.89,26.64 145.89,22.35 147,21.24 149.38,21.24 149.38,40.93 147.64,42.67 U1.24 | v127.16,32.04 128.11,31.08 130.81,31.08 v130.81,30.45
XTRA2  (via drill 0.35)
  Top 0.152: U1.P$22 U1.22 | v130.18,42.99 130.97,42.2 142.72,42.2 144.3,43.78 148.27,43.78 v148.59,43.47
  Bottom 0.152: GPIO.2 125.41,29.97 125.57,29.81 126.52,29.81 126.52,32.35 128.11,33.94 129.54,33.94 129.54,41.24 130.18,41.88 v130.18,42.99 | v148.59,43.47 148.43,43.62 148.43,46.64 U1.22
XTRA3  (via drill 0.35)
  Top 0.152: U1.25 U1.P$25 140.34,40.13 139.22,39.02 v135.73,39.02 | GPIO.1 123.03,28.54 123.67,28.54 123.98,28.86 126.84,28.86 127.16,28.54 127.79,28.54 128.11,28.86 v130.81,28.86
  Bottom 0.152: v130.81,28.86 131.44,29.5 131.44,34.73 v135.73,39.02

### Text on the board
tNames: IO | CLK | RX | TX | GND | 0 | 1 | picODE 3DO v1.2 | 2 | 3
